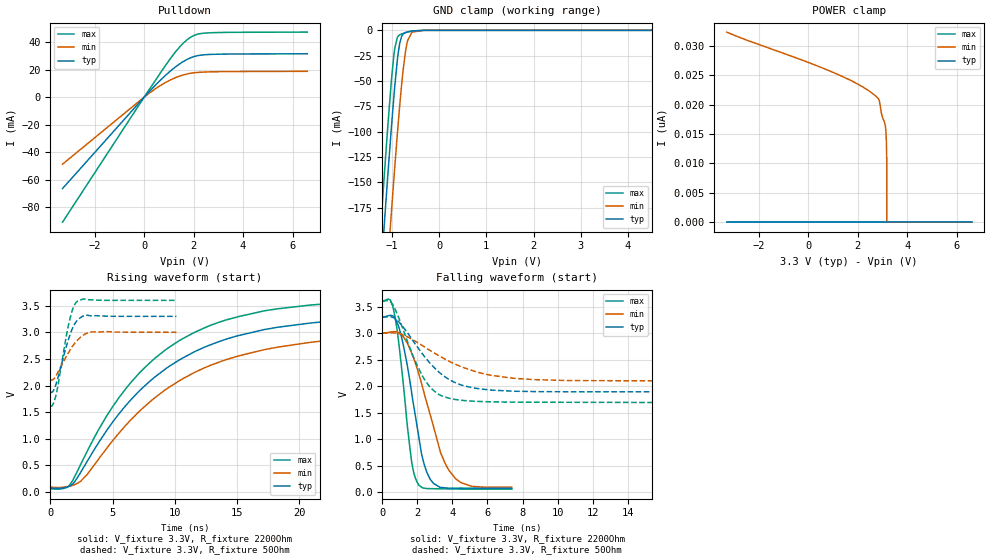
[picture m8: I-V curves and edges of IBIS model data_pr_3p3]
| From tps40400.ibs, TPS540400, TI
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|   data_pr_3p3 Model
[Model]   data_pr_3p3
Model_type   I/O_open_drain
Polarity   Inverting
Vinl = 0.8
Vinh = 2.1
Vmeas = 1.65
Vref = 3.3
Cref = 2pF
Rref = 2200
|   typ   min   max
|   (nom PVT)   (fast PVT)   (slow PVT)
C_comp   1.617e-12   1.585e-12   1.729e-12
| Where nom  PVT is Nominal Process, 3.3V, 25C
|   Fast PVT is Strong Process,  3.4V, -40C
|   Slow PVT is Weak Process,   3.2V, 125C
[Voltage Range]   3.3   3.2   3.4
|Junction Temperature
[Temperature Range]   25   125   -40
[Pullup Reference]   3.3   3.2   3.4
[Pulldown Reference]   0   0   0
[Power Clamp Reference]   3.3   3.2   3.4
[GND Clamp Reference]   0   0   0
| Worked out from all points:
|   slope of the pulldown table from 0 to 0.495 V, typ, clamps not added: 52.4 ohm
|   GND clamp passes 1 mA (typ) near -0.60 V on its own axis
|   falling waveform, V_fixture 3.3V, R_fixture 2200Ohm: 20-80 % time 971ps typ, 1.51ns min, 689ps max; typ from 3.3 V to 0.074 V
|   rising waveform, V_fixture 3.3V, R_fixture 2200Ohm: 20-80 % time 8.42ns typ, 9.22ns min, 7.76ns max; typ from 0.074 V to 3.3 V
|   falling waveform, V_fixture 3.3V, R_fixture 50Ohm: 20-80 % time 2.23ns typ, 3.22ns min, 1.6ns max; typ from 3.3 V to 1.88 V
|   rising waveform, V_fixture 3.3V, R_fixture 50Ohm: 20-80 % time 1.05ns typ, 1.37ns min, 905ps max; typ from 1.87 V to 3.3 V
[Pulldown]
|   Voltage   I(typ)   I(min)   I(max)
-3.3V     -66.53mA   -48.77mA   -91.01mA
257.4mV   5.028mA    3.596mA    6.933mA
814mV     15.05mA    10.18mA    21.76mA
1.253V    21.83mA    14.09mA    32.62mA
1.48V     24.77mA    15.62mA    37.4mA
1.756V    27.65mA    16.98mA    42.03mA
2.046V    29.71mA    17.82mA    45.17mA
2.439V    30.88mA    18.3mA     46.63mA
6.6V      31.61mA    18.84mA    47.39mA
[GND Clamp]
|   Voltage   I(typ)   I(min)   I(max)
-3.3V     -1.648A    -1.717A    -1.608A
-1.27V    -266.7mA   -355.3mA   -219.2mA
-1.165V   -195.4mA   -282.8mA   -146.8mA
-1.089V   -145.8mA   -231.9mA   -97.3mA
-1.009V   -95.8mA    -179.6mA   -49.55mA
-937mV    -54.97mA   -134.6mA   -17.46mA
-865.6mV  -22.65mA   -92.4mA    -5.675mA
-792mV    -6.034mA   -53.46mA   -3.563mA
-665mV    -1.602mA   -9.956mA   -1.625mA
-573.6mV  -736.5uA   -1.829mA   -633uA
-330.4mV  -7.166uA   -42.24uA   -2.454uA
6.6V      0A         0A         0A
[POWER Clamp]
|   Voltage   I(typ)   I(min)   I(max)
-3.3V     0A         32.36nA    0A
1.253V    0A         25.04nA    0A
2.153V    0A         23.15nA    0A
2.835V    0A         21.01nA    0A
2.886V    0A         20.41nA    0A
2.976V    0A         18.19nA    0A
3.103V    0A         16.67nA    0A
3.138V    0A         15.44nA    0A
3.158V    0A         13.55nA    0A
3.175V    0A         10.01nA    0A
3.177V    0A         0A         0A
6.6V      0A         0A         0A
[Ramp]
R_load = 2200
|   typ   min   max
dV/dt_r   1.93567/8.42941e-09   1.74469/9.24609e-09   2.12443/7.74739e-09
dV/dt_f   1.93578/9.6997e-10   1.74485/1.51031e-09   2.12452/6.88311e-10
[Falling Waveform]
V_fixture = 3.3V
V_fixture_min = 3V
V_fixture_max = 3.6V
R_fixture = 2200Ohm
|   Time   V(typ)   V(min)   V(max)
0s        3.3V       3V         3.6V
440ps     3.337V     3.022V     3.63V
660ps     3.31V      3.03V      3.413V
1.065ns   2.966V     2.98V      2.447V
1.67ns    1.882V     2.626V     578.9mV
2.085ns   1.034V     2.228V     133.6mV
2.73ns    245.5mV    1.464V     69.77mV
3.325ns   92.78mV    745.7mV    66.21mV
4.175ns   78.19mV    257.9mV    62.36mV
7.385ns   74.32mV    96.3mV     59.17mV
[Rising Waveform]
V_fixture = 3.3V
V_fixture_min = 3V
V_fixture_max = 3.6V
R_fixture = 2200Ohm
|   Time   V(typ)   V(min)   V(max)
0s        73.69mV    91.87mV    59.13mV
1.57ns    114.5mV    110.4mV    133.5mV
2.97ns    578.9mV    330.1mV    768.6mV
4.635ns   1.192V     852.9mV    1.467V
7.41ns    1.956V     1.571V     2.296V
10.3ns    2.471V     2.08V      2.834V
13.82ns   2.848V     2.462V     3.21V
18.25ns   3.094V     2.721V     3.441V
24.99ns   3.243V     2.898V     3.567V
46.16ns   3.298V     2.995V     3.599V
[Falling Waveform]
V_fixture = 3.3V
V_fixture_min = 3V
V_fixture_max = 3.6V
R_fixture = 50Ohm
|   Time   V(typ)   V(min)   V(max)
0s        3.3V       3V         3.6V
390ps     3.311V     3.007V     3.61V
625ps     3.296V     3.006V     3.522V
2ns       2.741V     2.826V     2.384V
2.85ns    2.39V      2.649V     1.942V
4.195ns   2.063V     2.412V     1.75V
6.06ns    1.933V     2.217V     1.707V
8.725ns   1.899V     2.125V     1.699V
15.77ns   1.896V     2.102V     1.694V
200ns     1.876V     2.104V     1.625V
[Rising Waveform]
V_fixture = 3.3V
V_fixture_min = 3V
V_fixture_max = 3.6V
R_fixture = 50Ohm
|   Time   V(typ)   V(min)   V(max)
0s        1.87V      2.104V     1.611V
205ps     1.888V     2.109V     1.642V
430ps     2.004V     2.171V     1.793V
650ps     2.178V     2.263V     2.042V
1.465ns   2.869V     2.618V     3.138V
1.805ns   3.086V     2.744V     3.437V
2.115ns   3.21V      2.835V     3.571V
2.71ns    3.313V     2.955V     3.624V
3.43ns    3.312V     3.009V     3.61V
10.14ns   3.3V       3V         3.6V
